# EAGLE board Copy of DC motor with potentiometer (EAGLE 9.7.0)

Size 251.73 x 98.71 mm. Coordinates in mm from the lower left corner, seen from the top.
Outline: 0,0 251.73,0 251.73,98.71 0,98.71 0,0
Copper layers (1*16): Top 0.035mm / dielectric 1.5mm / Bottom 0.035mm
Design rules "default": minimum track width 6mil, minimum drill 0.35mm, track to track 6mil, track to pad 6mil, pad to pad 6mil, via to via 6mil, smd to smd 6mil, copper to edge 40mil, drill to drill 6mil, minimum pad ring 10mil, minimum via ring 8mil, stop-mask expansion 4mil, vias tented up to drill 0mil, thermal gap 10mil

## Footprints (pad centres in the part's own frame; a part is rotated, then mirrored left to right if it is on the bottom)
BATTERY-GENERIC = drill 1.118 pad 3.15 octagon: + 2.54,0; - -2.54,0
DG01D = drill 1.118 pad 3.15 octagon: + 2.54,0; - -2.54,0
HA-06-SM065 = drill 1 pad 1.676: 1 -2.54,-2.54; 2 0,2.54; 3 2.54,-2.54
ARDUINO-UNO-R3-SHIELD = drill 1.016 pad 1.88: 3.3V 24.13,-2.54; 5V 24.13,0; A0 24.13,12.7; A1 24.13,15.24; A2 24.13,17.78; A3 24.13,20.32; A4 24.13,22.86; A5 24.13,25.4; AREF -24.13,-13.97; D2 -24.13,20.32; D3 -24.13,17.78; D4 -24.13,15.24; D5 -24.13,12.7; D6 -24.13,10.16; D7 -24.13,7.62; D8 -24.13,3.81; D9 -24.13,1.27; D10 -24.13,-1.27; D11 -24.13,-3.81; D12 -24.13,-6.35; D13 -24.13,-8.89; GND@0 24.13,2.54; GND@1 24.13,5.08; GND@2 -24.13,-11.43; IOREF 24.13,-7.62; NC 24.13,-10.16; RES 24.13,-5.08; RX -24.13,25.4; SCL -24.13,-19.05; SDA -24.13,-16.51; TX -24.13,22.86; VIN 24.13,7.62

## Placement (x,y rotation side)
BAT1  9V  [BATTERY-GENERIC]  243.47,39.1 180 top
M2  MOTOR_DG01D  [DG01D]  201.86,86.01 270 top
RPOT1  250k  [HA-06-SM065]  184.01,16.85 0 top
U1  ARDUINO-UNO-R3-SHIELD  [ARDUINO-UNO-R3-SHIELD]  47.88,29.84 270 top

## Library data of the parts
BAT1 M2 RPOT1 U1 = Tinkercad

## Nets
BAT1+: BAT1.+ M2.+
BAT1-: BAT1.- RPOT1.1 U1.GND@0 U1.GND@1 U1.GND@2
U1_5V: RPOT1.3 U1.5V
U1_A0: RPOT1.2 U1.A0

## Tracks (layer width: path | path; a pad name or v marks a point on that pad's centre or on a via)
BAT1+  (1 unrouted)
BAT1-  (4 unrouted)
U1_5V  (1 unrouted)
U1_A0  (1 unrouted)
